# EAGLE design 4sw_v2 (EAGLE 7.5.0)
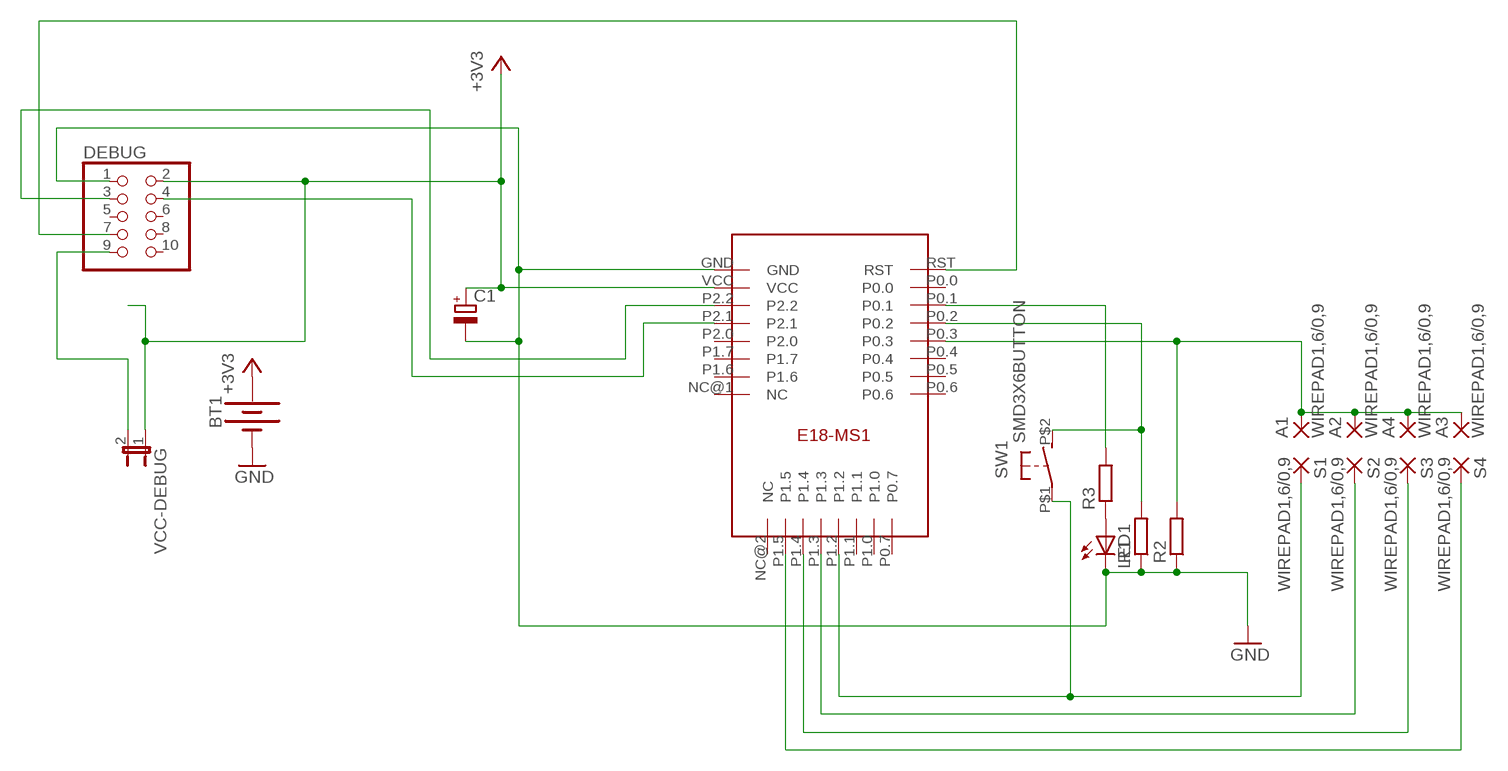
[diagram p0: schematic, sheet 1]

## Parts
A1  WIREPAD1,6/0,9  [1,6/0,9]
A2  WIREPAD1,6/0,9  [1,6/0,9]
A3  WIREPAD1,6/0,9  [1,6/0,9]
A4  WIREPAD1,6/0,9  [1,6/0,9]
BT1  BATTERY-20MM_SMD_4LEGS  [BATTCON_20MM_4LEGS]
C1  CPOL-EUSMCD  [SMC_D]
DEBUG  PINHD-2X5  [2X05]
LED1  LEDSML0805  [SML0805]
R1  R-EU_R0805  [R0805]
R2  R-EU_R0805  [R0805]
R3  R-EU_M0805  [M0805]
S1  WIREPAD1,6/0,9  [1,6/0,9]
S2  WIREPAD1,6/0,9  [1,6/0,9]
S3  WIREPAD1,6/0,9  [1,6/0,9]
S4  WIREPAD1,6/0,9  [1,6/0,9]
SW1  SMD3X6BUTTON  [SMD3X6]
U$1  E18-MS1PCB  [E18-MS1-PCB]
VCC-DEBUG  JP1E  [JP1]

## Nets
+3V3: BT1.POSITIVE@1(+) BT1.POSITIVE@2(+) BT1.POSITIVE@3(+) BT1.POSITIVE@4(+) C1.+ DEBUG.2 U$1.VCC VCC-DEBUG.1
GND: BT1.NEGATIVE(-) C1.- DEBUG.1 LED1.C R1.1 R2.1 U$1.GND
N$1: R1.2 SW1.P$2(S) U$1.P0.2
N$2: S1.1(P) SW1.P$1(P) U$1.P1.2
N$3: S2.1(P) U$1.P1.3
N$4: DEBUG.9 VCC-DEBUG.2
N$7: R3.2 U$1.P0.1
N$8: LED1.A R3.1
N$10: S3.1(P) U$1.P1.4
N$11: S4.1(P) U$1.P1.5
N$12: DEBUG.7 U$1.RST
N$13: DEBUG.3 U$1.P2.2
N$14: DEBUG.4 U$1.P2.1
N$17: A1.1(P) A2.1(P) A3.1(P) A4.1(P) R2.2 U$1.P0.3
Unconnected: DEBUG.5 DEBUG.6 DEBUG.8 DEBUG.10 U$1.NC@1(NC) U$1.NC@2(NC) U$1.P0.0 U$1.P0.4 U$1.P0.5 U$1.P0.6 U$1.P0.7 U$1.P1.0 U$1.P1.1 U$1.P1.6 U$1.P1.7 U$1.P2.0

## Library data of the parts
A1-A4 S1-S4 = wirepad:WIREPAD: Wire PAD connect wire on PCB
BT1 = SparkFun-Batteries:BATTERY: Battery - Single Cell; PROD_ID: BATT-10373; SF_SKU: PRT-11892
C1 = resistor:CPOL-EU: POLARIZED CAPACITOR, European symbol
DEBUG = pinhead:PINHD-2X5: PIN HEADER
LED1 = led:LED: LED
R1-R3 = resistor:R-EU_: RESISTOR, European symbol
SW1 = andi:SMD3X6BUTTON
U$1 = e18-ms1-ipx-pcb:E18-MS1
VCC-DEBUG = jumper:JP1E: JUMPER

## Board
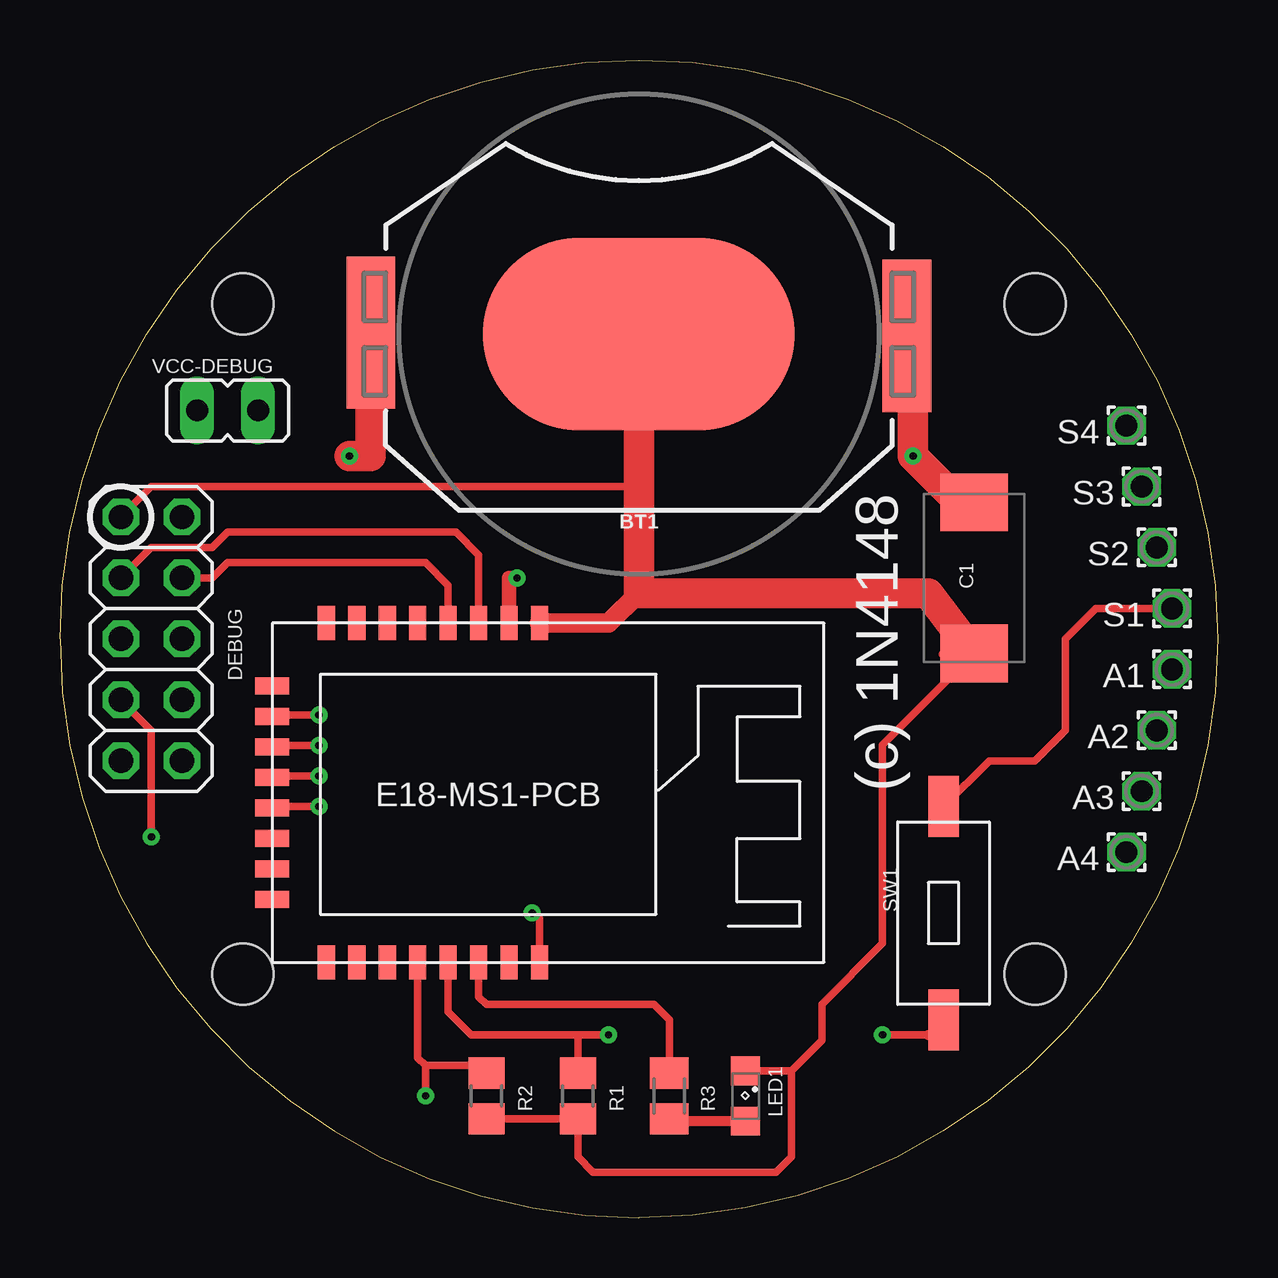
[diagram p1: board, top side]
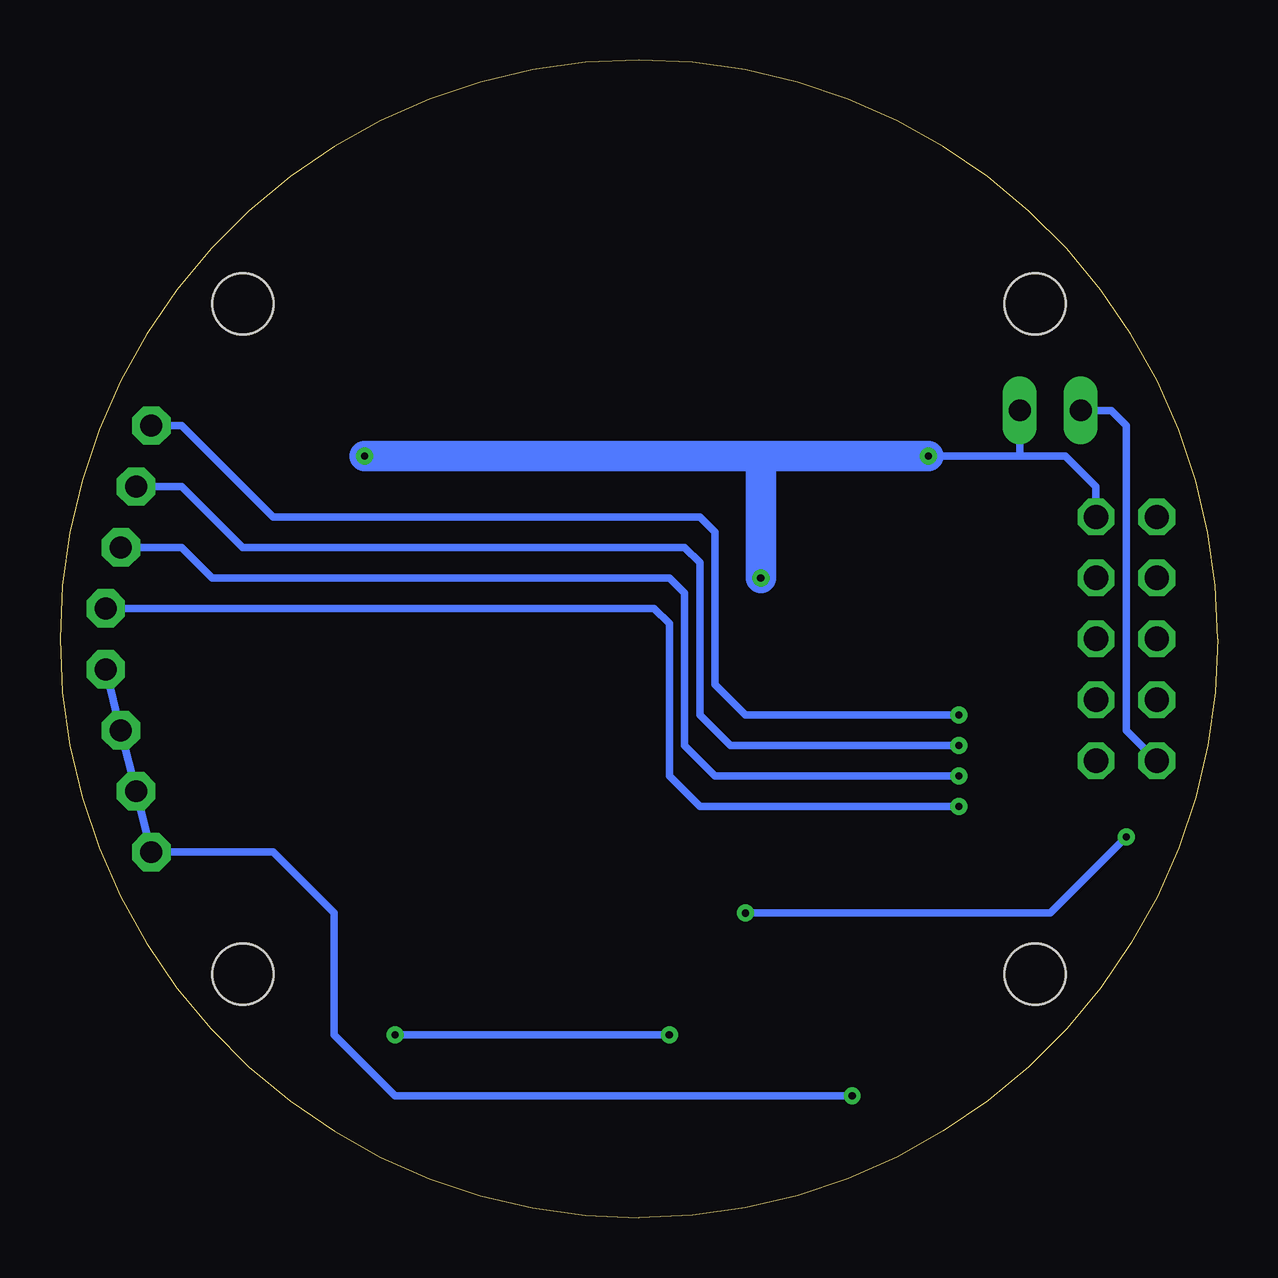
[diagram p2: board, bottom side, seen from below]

Size 48.26 x 48.26 mm. Coordinates in mm from the lower left corner, seen from the top.
Outline: 0,24.13 arc90 24.13,0 arc90 48.26,24.13 arc90 24.13,48.26 arc90 0,24.13
Copper layers (1*16): Top 0.035mm / dielectric 1.5mm / Bottom 0.035mm
Design rules "default": minimum track width 10mil, minimum drill 24mil, track to track 8mil, track to pad 8mil, pad to pad 8mil, via to via 8mil, smd to smd 8mil, copper to edge 40mil, drill to drill 8mil, minimum pad ring 10mil, minimum via ring 8mil, stop-mask expansion 4mil, vias tented up to drill 0mil, thermal gap 10mil
Holes 2.54 mm at 7.62,38.1 40.64,38.1 40.64,10.16 7.62,10.16

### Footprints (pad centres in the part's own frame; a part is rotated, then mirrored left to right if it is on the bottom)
1,6/0,9 = drill 0.914 pad 1.6 octagon: 1 0,0
BATTCON_20MM_4LEGS = smd 13 x 8: NEGATIVE 0,0 | smd 2.032 x 3.175: POSITIVE@1 -11.176,1.651; POSITIVE@2 -11.176,-1.524; POSITIVE@3 11.176,1.524; POSITIVE@4 11.176,-1.651
SMC_D = smd 2.4 x 2.8: + -3.15,0; - 3.15,0
2X05 = drill 1.016 octagon: 1 -5.08,-1.27; 2 -5.08,1.27; 3 -2.54,-1.27; 4 -2.54,1.27; 5 0,-1.27; 6 0,1.27; 7 2.54,-1.27; 8 2.54,1.27; 9 5.08,-1.27; 10 5.08,1.27
SML0805 = smd 1.2 x 1.2: A 1.05,0; C -1.05,0
R0805 = smd 1.3 x 1.5: 1 -0.95,0; 2 0.95,0
M0805 = smd 1.3 x 1.6: 1 -0.95,0; 2 0.95,0
SMD3X6 = smd 2.54 x 1.27: P$1 4.445,0; P$2 -4.445,0
E18-MS1-PCB = smd 0.711 x 1.422: GND 11.15,14.14; NC@1 2.26,14.14; P0.0 9.88,0; P0.1 8.61,0; P0.2 7.34,0; P0.3 6.07,0; P0.4 4.8,0; P0.5 3.53,0; P0.6 2.26,0; P1.6 3.53,14.14; P1.7 4.8,14.14; P2.0 6.07,14.14; P2.1 7.34,14.14; P2.2 8.61,14.14; RST 11.15,0; VCC 9.88,14.14 | smd 1.422 x 0.711: NC@2 0,11.51; P0.7 0,2.62; P1.0 0,3.89; P1.1 0,5.16; P1.2 0,6.43; P1.3 0,7.7; P1.4 0,8.97; P1.5 0,10.24
JP1 = drill 0.914 long: 1 0,-1.27; 2 0,1.27

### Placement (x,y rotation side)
A1  46.35,22.86 0 top
A2  45.72,20.32 0 top
A3  45.09,17.78 0 top
A4  44.45,15.24 0 top
BT1  24.13,36.83 180 top
C1  38.1,26.67 270 top
DEBUG  3.81,24.13 270 top
LED1  28.57,5.08 270 top
R1  21.59,5.08 90 top
R2  17.78,5.08 90 top
R3  25.4,5.08 90 top
S1  46.35,25.4 0 top
S2  45.72,27.94 0 top
S3  45.09,30.48 0 top
S4  44.45,33.02 0 top
SW1  36.83,12.7 90 top
U$1  8.85,10.65 0 top
VCC-DEBUG  6.99,33.66 90 top

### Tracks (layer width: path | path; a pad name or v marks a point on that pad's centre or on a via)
+3V3  (via drill 0.3 pad 0.4)
  Top 0.406: BT1.POSITIVE@3 BT1.POSITIVE@4 | BT1.POSITIVE@2 BT1.POSITIVE@1
  Top 0.61: U$1.VCC 18.73,26.67 v19.05,26.67 | 35.56,35.18 BT1.POSITIVE@1 | BT1.POSITIVE@3 12.95,34.04
  Top 0.813: C1.+ 37.49,29.82
  Top 1.27: 35.56,35.18 v35.56,31.75 37.49,29.82 | v12.06,31.75 12.95,31.75 BT1.POSITIVE@3
  Bottom 0.305: v12.06,31.75 8.26,31.75 | 8.26,31.75 6.35,31.75 5.08,30.48 DEBUG.2 | VCC-DEBUG.1 8.26,31.75
  Bottom 1.27: v19.05,26.67 19.05,31.75 | 19.05,31.75 v35.56,31.75 | v12.06,31.75 19.05,31.75
GND
  Top 0.305: R2.1 R1.1 21.59,2.54 22.23,1.91 29.84,1.91 30.48,2.54 30.48,6.13 | LED1.C 30.48,6.13 | 30.48,6.13 31.75,7.4 31.75,8.89 34.29,11.43 34.29,19.71 C1.- | DEBUG.1 3.81,30.48 24.13,30.48
  Top 0.406: 36.83,23.5 C1.-
  Top 0.813: 24.13,26.05 arc-90 24.13,26.05 22.87,24.79 U$1.GND
  Top 1.27: 24.13,26.05 24.13,30.48 BT1.NEGATIVE | C1.- 36.2,26.01 24.13,26.05
N$1  (via drill 0.3 pad 0.4)
  Top 0.305: U$1.P0.2 16.18,8.58 17.14,7.62 21.59,7.62 | R1.2 21.59,7.62 | 21.59,7.62 v22.86,7.62 | v34.29,7.62 36.2,7.62
  Top 0.406: 36.2,7.62 arc90 SW1.P$2
  Bottom 0.305: v22.86,7.62 v34.29,7.62
N$2  (via drill 0.3 pad 0.4)
  Top 0.305: U$1.P1.2 8.91,17.14 v10.79,17.14 | S1.1 43.18,25.4 41.91,24.13 41.91,20.32 40.64,19.05 38.73,19.05 SW1.P$1
  Bottom 0.305: S1.1 23.5,25.4 22.86,24.77 22.86,18.41 21.59,17.14 v10.79,17.14
N$3  (via drill 0.3 pad 0.4)
  Top 0.305: U$1.P1.3 8.91,18.41 v10.79,18.41
  Bottom 0.305: S2.1 43.18,27.94 41.91,26.67 22.86,26.67 22.23,26.04 22.23,19.68 20.95,18.41 v10.79,18.41
N$4
  Bottom 0.305: DEBUG.9 3.81,20.32 3.81,33.02 4.45,33.66 VCC-DEBUG.2
N$7
  Top 0.305: U$1.P0.1 17.45,9.21 17.78,8.89 24.77,8.89 25.4,8.26 R3.2
N$8
  Top 0.406: LED1.A 25.5,4.03 R3.1
N$10  (via drill 0.3 pad 0.4)
  Top 0.305: U$1.P1.4 8.91,19.68 v10.79,19.68
  Bottom 0.305: S3.1 43.18,30.48 40.64,27.94 22.23,27.94 21.59,27.3 21.59,20.95 20.32,19.68 v10.79,19.68
N$11  (via drill 0.3 pad 0.4)
  Top 0.305: U$1.P1.5 8.91,20.95 v10.79,20.95
  Bottom 0.305: S4.1 43.18,33.02 39.37,29.21 21.59,29.21 20.95,28.57 20.95,22.23 19.68,20.95 v10.79,20.95
N$12  (via drill 0.3 pad 0.4)
  Top 0.305: v3.81,15.88 3.81,20.32 DEBUG.7 | U$1.RST 20,12.39 arc90 v19.68,12.7
  Bottom 0.305: v19.68,12.7 6.99,12.7 v3.81,15.88
N$13
  Top 0.305: U$1.P2.2 17.45,27.63 16.51,28.57 6.99,28.57 6.35,27.94 3.81,27.94 DEBUG.3
N$14
  Top 0.305: U$1.P2.1 16.18,26.36 15.24,27.3 6.99,27.3 6.35,26.67 DEBUG.4
N$17  (via drill 0.3 pad 0.4)
  Top 0.305: U$1.P0.3 14.91,6.67 15.24,6.35 | 15.24,6.35 17.46,6.35 | v15.24,5.08 15.24,6.35
  Top 0.406: 17.46,6.35 R2.2
  Bottom 0.305: A1.1 A2.1 A3.1 A4.1 39.37,15.24 36.83,12.7 36.83,7.62 34.29,5.08 v15.24,5.08

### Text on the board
tNames: (c) 1N4148

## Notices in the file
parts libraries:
SparkFun-Batteries: Licensing: Creative Commons ShareAlike 4.0 International - https://creativecommons.org/licenses/by-sa/4.0
